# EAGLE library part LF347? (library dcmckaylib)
Quad FET Op-Amp with 4MHz Bandwidth Low input bias current Moderate voltage noise and input voltage offset
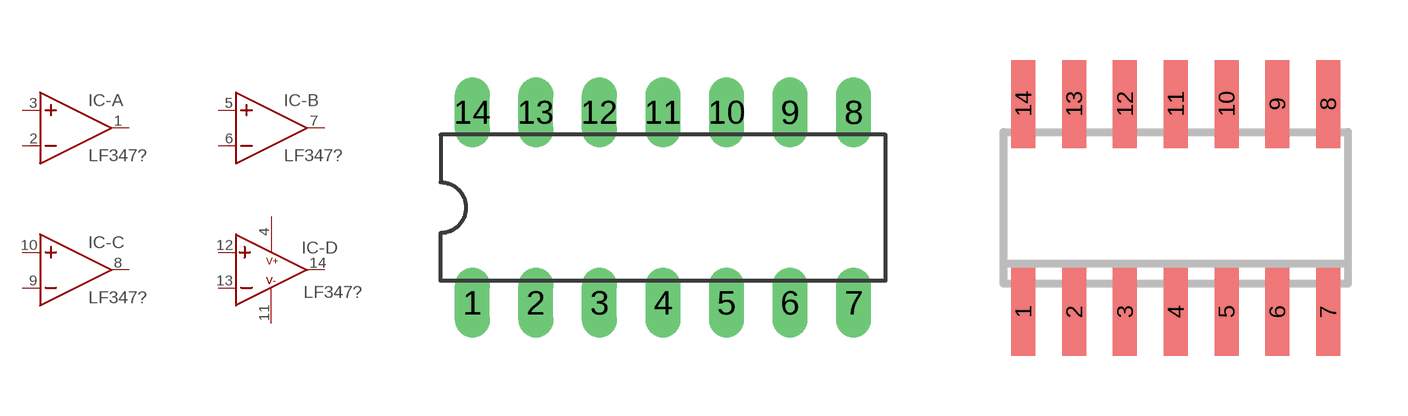
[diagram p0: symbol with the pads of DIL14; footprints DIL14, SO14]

Designator prefix IC; gates -A=OPAMP -B=OPAMP -C=OPAMP -D=OPAMP2

## LF347N  [DIL14]
1  -A:OUT  out
2  -A:IN-  in
3  -A:IN+  in
4  -D:V+  pwr
5  -B:IN+  in
6  -B:IN-  in
7  -B:OUT  out
8  -C:OUT  out
9  -C:IN-  in
10  -C:IN+  in
11  -D:V-  pwr
12  -D:IN+  in
13  -D:IN-  in
14  -D:OUT  out

## LF347D  [SO14]
Pads as for DIL14

## Footprint DIL14 (pad centres in mm)
Dual In Line Package
drill 0.889 long: 1 -7.62,-3.81; 2 -5.08,-3.81; 3 -2.54,-3.81; 4 0,-3.81; 5 2.54,-3.81; 6 5.08,-3.81; 7 7.62,-3.81; 8 7.62,3.81; 9 5.08,3.81; 10 2.54,3.81; 11 0,3.81; 12 -2.54,3.81; 13 -5.08,3.81; 14 -7.62,3.81

## Footprint SO14 (pad centres in mm)
Small Outline Package 14
smd 0.6 x 2.2: 1 -3.81,-2.6; 2 -2.54,-2.6; 3 -1.27,-2.6; 4 0,-2.6; 5 1.27,-2.6; 6 2.54,-2.6; 7 3.81,-2.6; 8 3.81,2.6; 9 2.54,2.6; 10 1.27,2.6; 11 0,2.6; 12 -1.27,2.6; 13 -2.54,2.6; 14 -3.81,2.6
